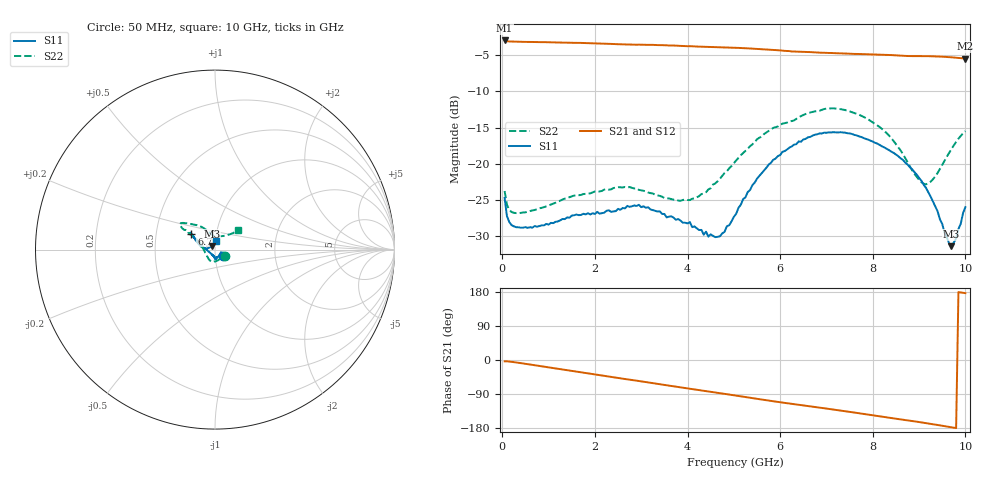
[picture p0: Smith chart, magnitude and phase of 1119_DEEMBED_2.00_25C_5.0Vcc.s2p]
!Hittite Microwave Corp.
!Digital Attenuator/PhaseShifter Rev 1.4.0
!Filename: C:\DATA\DATA\1119_DEEMBED_2.00_25C_5.0Vcc.s2p
!VNA ID: Agilent Technologies,N5224A,MY51441122,A.10.45.03
!Device type:
!2 Port Calibration.
!Temp(C): 25
!Lot Number:
!Serial Number:
!Operator:
!Misc:
!Attenuator:  2.000
# GHZ S DB R 50.0
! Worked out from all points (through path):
!   200 points, 50 MHz to 10 GHz, reference 50 ohm
!   highest |S21| = -2.95 dB at 50 MHz (marker M1); lowest = -5.4 dB at 10 GHz (marker M2)
!   group delay of S21, straight-line fit = 50.2 ps
!   lowest |S11| = -31.4 dB at 9.7 GHz (marker M3), VSWR 1.06, Z = 48.2 + j1.92 ohm
!   |S11| at or under -10 dB: start of sweep to end of sweep
!   |S22| runs from -26.8 to -12.3 dB; largest |S21 - S12| = 0.0018
!   S11 on the Smith chart (normalised r, x): 50 MHz: 1.09, -0.08; 6.75 GHz: 0.76, +0.14; 10 GHz: 1.01, +0.10
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0.05  -24.72 -37.1  -2.95 -3.6  -2.94 -3.6  -23.76 -30.4
0.1  -27.20 -29.6  -3.06 -3.5  -3.05 -3.5  -25.65 -24.7
0.15  -28.04 -25.7  -3.09 -4.0  -3.09 -4.0  -26.35 -22.0
0.3  -28.76 -23.1  -3.12 -6.4  -3.12 -6.5  -26.81 -22.2
1.75  -26.90 -74.8  -3.30 -33.5  -3.30 -33.5  -24.18 -74.5
2.75  -25.95 -85.3  -3.52 -51.9  -3.52 -52.0  -23.21 -108.8
3.4  -26.56 -92.5  -3.59 -63.8  -3.60 -63.9  -24.43 -131.7
4.05  -28.04 -99.1  -3.74 -75.8  -3.75 -75.8  -25.01 -160.9
4.6  -30.13 -132.2  -3.88 -85.8  -3.89 -85.8  -22.70 166.5
4.8  -29.39 -154.8  -3.91 -89.4  -3.93 -89.4  -21.27 158.8
5.05  -26.91 -176.3  -3.97 -94.0  -3.99 -94.0  -19.55 152.6
5.4  -22.95 166.9  -4.08 -100.6  -4.09 -100.6  -17.31 149.5
5.85  -19.45 156.5  -4.26 -108.8  -4.28 -108.9  -15.03 147.1
6.7  -16.10 146.6  -4.58 -123.2  -4.59 -123.2  -12.82 145.8
6.75  -15.98 145.9  -4.60 -124.1  -4.61 -124.1  -12.75 145.5
7.5  -15.79 146.4  -4.78 -137.0  -4.79 -137.0  -12.75 139.8
8.35  -18.10 152.4  -4.96 -152.2  -4.96 -152.2  -16.09 123.0
9.15  -23.32 171.8  -5.12 -166.5  -5.13 -166.5  -22.83 84.2
9.35  -25.91 173.8  -5.15 -170.4  -5.16 -170.5  -21.73 64.7
9.7  -31.38 132.5  -5.28 -177.6  -5.29 -177.6  -17.95 44.0
9.799999  -30.33 107.2  -5.33 -179.7  -5.34 -179.7  -16.97 42.0
10  -25.98 83.2  -5.45 176.3  -5.46 176.3  -15.48 39.9
